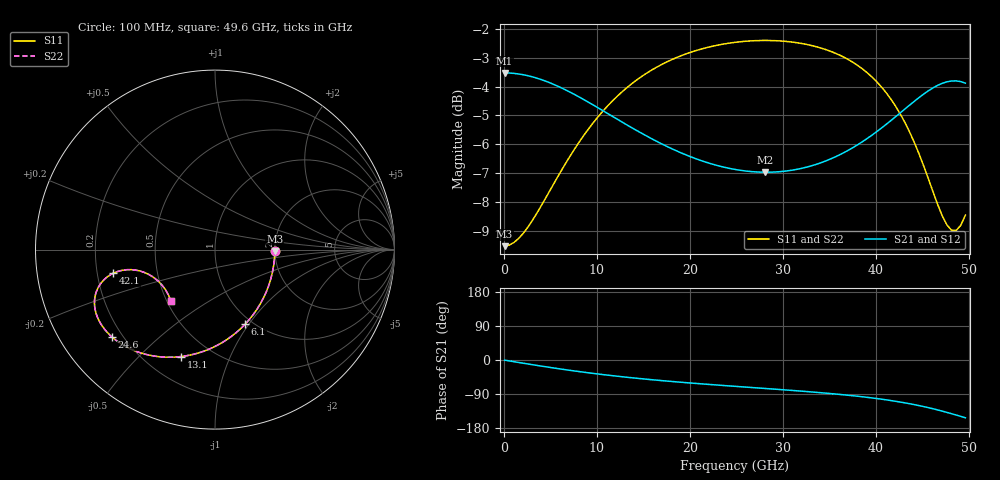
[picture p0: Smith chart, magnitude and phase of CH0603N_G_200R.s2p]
# GHz S RI R 200
! S-Parameters data
! Freq  reS11  imS11  reS21  imS21  reS12  imS12  reS22  imS22
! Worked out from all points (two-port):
!   100 points, 100 MHz to 49.6 GHz, reference 200 ohm
!   highest |S21| = -3.52 dB at 100 MHz (marker M1); lowest = -7.0 dB at 28.1 GHz (marker M2)
!   |S21| within 3 dB of the highest: start of sweep to 20.81 GHz; 35.04 GHz to end of sweep
!   lowest |S11| = -9.5 dB at 100 MHz (marker M3), VSWR 2.00, Z = 400 - j7.07 ohm
!   |S11| at or under -10 dB: nowhere
!   |S22| runs from -9.5 to -2.4 dB; largest |S21 - S12| = 0
!   S11 on the Smith chart (normalised r, x): 100 MHz: 2.00, -0.04; 6.1 GHz: 0.92, -0.96; 13.1 GHz: 0.34, -0.67; 24.6 GHz: 0.16, -0.36; 42.1 GHz: 0.27, -0.11; 49.6 GHz: 0.52, -0.35
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0.1  0.3333 -0.00785  0.6666 -0.00471  0.6666 -0.00471  0.3333 -0.00785
1.6  0.3204 -0.1244  0.6596 -0.0747  0.6596 -0.0747  0.3204 -0.1244
3.1  0.2862 -0.2343  0.6407 -0.141  0.6407 -0.141  0.2862 -0.2343
6.1  0.1678 -0.4158  0.576 -0.2526  0.576 -0.2526  0.1678 -0.4158
8.6  0.0408 -0.5174  0.5072 -0.3191  0.5072 -0.3191  0.0408 -0.5174
10.6  -0.0649 -0.567  0.4503 -0.3557  0.4503 -0.3557  -0.0649 -0.567
13.1  -0.1905 -0.596  0.3828 -0.3853  0.3828 -0.3853  -0.1905 -0.596
16.6  -0.3424 -0.5925  0.3003 -0.4066  0.3003 -0.4066  -0.3424 -0.5925
20.6  -0.4765 -0.5508  0.2241 -0.4168  0.2241 -0.4168  -0.4765 -0.5508
24.6  -0.5723 -0.4883  0.1625 -0.4238  0.1625 -0.4238  -0.5723 -0.4883
25.1  -0.5819 -0.4796  0.1554 -0.4249  0.1554 -0.4249  -0.5819 -0.4796
28.1  -0.6291 -0.4245  0.1149 -0.4331  0.1149 -0.4331  -0.6291 -0.4245
33.1  -0.6696 -0.3234  0.0451 -0.4577  0.0451 -0.4577  -0.6696 -0.3234
37.6  -0.657 -0.2241  -0.0392 -0.4938  -0.0392 -0.4938  -0.657 -0.2241
39.6  -0.6297 -0.18  -0.0922 -0.512  -0.0922 -0.512  -0.6297 -0.18
41.6  -0.5834 -0.1406  -0.1612 -0.5268  -0.1612 -0.5268  -0.5834 -0.1406
42.1  -0.5684 -0.1324  -0.1815 -0.5291  -0.1815 -0.5291  -0.5684 -0.1324
44.1  -0.4927 -0.1121  -0.2768 -0.5265  -0.2768 -0.5265  -0.4927 -0.1121
46.1  -0.3956 -0.1264  -0.3914 -0.4906  -0.3914 -0.4906  -0.3956 -0.1264
48.1  -0.2967 -0.1958  -0.5059 -0.4007  -0.5059 -0.4007  -0.2967 -0.1958
48.6  -0.2763 -0.2228  -0.53 -0.3687  -0.53 -0.3687  -0.2763 -0.2228
49.6  -0.2457 -0.2866  -0.5676 -0.2952  -0.5676 -0.2952  -0.2457 -0.2866
